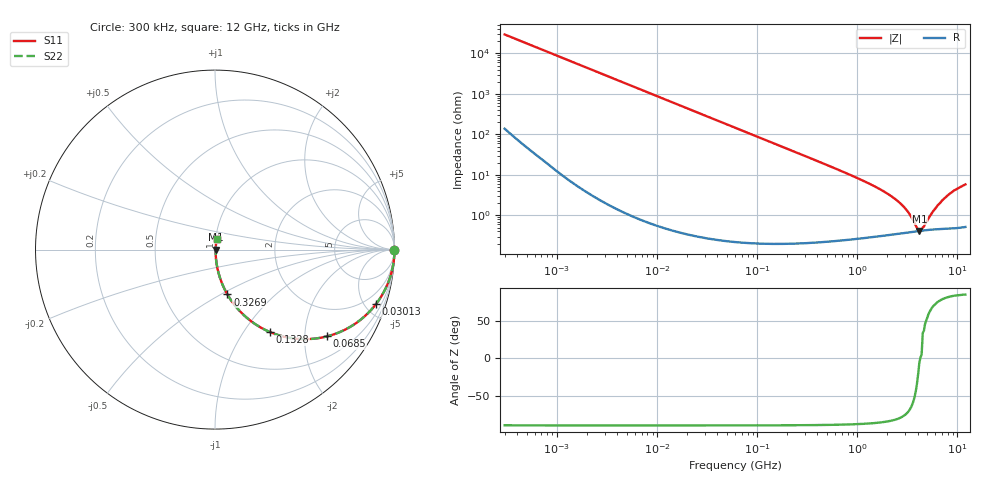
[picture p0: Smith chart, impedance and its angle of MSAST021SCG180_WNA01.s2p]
! MSAST021SCG180_WNA01  S-PARAMETER MODEL  ( General Type )
! Model Generated by TAIYO YUDEN Corporation (http://www.ty-top.com)
! Version 2.0
! TAIYO YUDEN Control No. 181101
! Copyright(c) 2016 TAIYO YUDEN CO.,LTD. All Rights Reserved.
! Product Description (link to TY-COMPAS)
! https://ds.yuden.co.jp/TYCOMPAS/or/detail?pn=MSAST021SCG180JWNA01&u=M
! Products Name : Multilayer Ceramic Capacitors
! Characteristics :
!  Capacitance : 18 pF , Rated Voltage : 25V , TCC : CG / C0G
!  Case Size : 0.25 x 0.125 / 0.0098 x 0.0049 [mm/inch] , Thickness : 0.125 / 0.0049 [mm/inch]
!  (Conditions: Temperature = 25 degC , DC Bias Current/Voltage = 0A / 0V)
! External Node Assignments :
!  1  o---| |---o  2
! GND o---------o GND
! Frequency Range : 0.3MHz  -  12000MHz  [ 401 STEP ]
# MHz S RI R 50
! Freq[MHz].  S11 Real  S11 Imag  S21 Real  S21 Imag  S12 Real  S12 Imag  S22 Real  S22 Imag
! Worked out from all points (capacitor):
!   401 points, 300 kHz to 12 GHz, reference 50 ohm
!   read as one part in series: C = 18 pF near 316.3 kHz
!   lowest |Z| = 414 mohm at 4.159 GHz (marker M1)
!   series resonance near 4.257 GHz, so ESL is about 78 pH
!   S11 on the Smith chart (normalised r, x): 300 kHz: open; 30.13 MHz: 1.01, -5.87; 68.5 MHz: 1.00, -2.58; 132.8 MHz: 1.00, -1.33; 326.9 MHz: 1.00, -0.54; 12 GHz: 1.01, +0.12
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0.3  1 -0.00339  2.74e-05 0.00339  2.74e-05 0.00339  1 -0.00339
1.769972  0.9996 -0.02  0.000418 0.02  0.000418 0.02  0.9996 -0.02
10.44266  0.9862 -0.1165  0.0138 0.1165  0.0138 0.1165  0.9862 -0.1165
30.13126  0.8957 -0.3052  0.1043 0.3052  0.1043 0.3052  0.8957 -0.3052
60  0.6844 -0.464  0.3156 0.464  0.3156 0.464  0.6844 -0.464
68.49786  0.6246 -0.4834  0.3754 0.4834  0.3754 0.4834  0.6246 -0.4834
94.13233  0.4686 -0.4979  0.5314 0.4979  0.5314 0.4979  0.4686 -0.4979
132.8329  0.3071 -0.4598  0.6929 0.4598  0.6929 0.4598  0.3071 -0.4598
202.9496  0.16 -0.3644  0.84 0.3644  0.84 0.3644  0.16 -0.3644
326.9496  0.0691 -0.2497  0.9309 0.2497  0.9309 0.2497  0.0691 -0.2497
353.9943  0.0597 -0.2327  0.9403 0.2327  0.9403 0.2327  0.0597 -0.2327
1105.905  0.00816 -0.0736  0.9918 0.0736  0.9918 0.0736  0.00816 -0.0736
2088.533  0.00426 -0.0317  0.9957 0.0317  0.9957 0.0317  0.00426 -0.0317
3026.31  0.00387 -0.014  0.9961 0.014  0.9961 0.014  0.00387 -0.014
3364.605  0.0039 -0.00939  0.9961 0.00939  0.9961 0.00939  0.0039 -0.00939
3944.255  0.00403 -0.00268  0.996 0.00268  0.996 0.00268  0.00403 -0.00268
4158.869  0.00409 -0.000466  0.9959 0.000466  0.9959 0.000466  0.00409 -0.000466
4502.883  0.0042 0.0028  0.9958 -0.0028  0.9958 -0.0028  0.0042 0.0028
5715.274  0.00459 0.0117  0.9954 -0.0117  0.9954 -0.0117  0.00459 0.0117
7254.098  0.0052 0.0244  0.9948 -0.0244  0.9948 -0.0244  0.0052 0.0244
9207.246  0.00636 0.04  0.9936 -0.04  0.9936 -0.04  0.00636 0.04
12000  0.00842 0.0571  0.9916 -0.0571  0.9916 -0.0571  0.00842 0.0571
